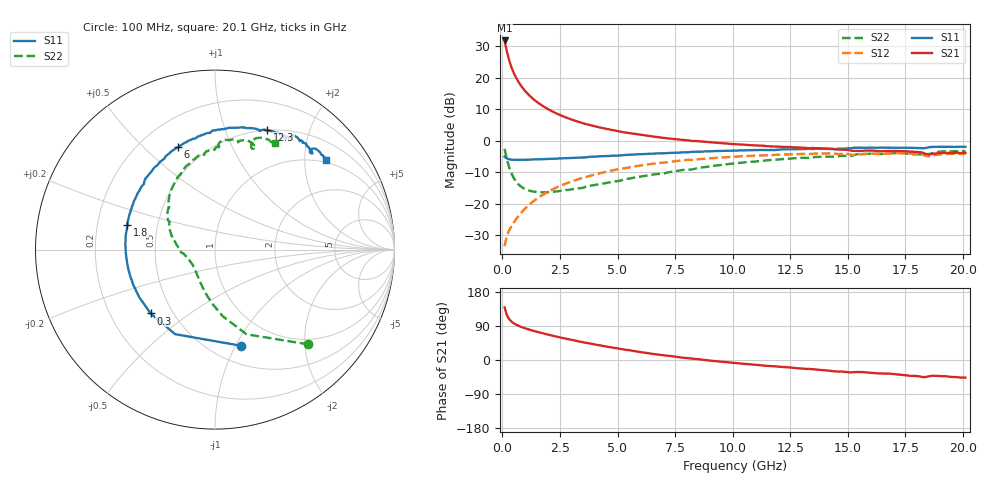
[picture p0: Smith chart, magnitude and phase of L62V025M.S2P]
!  Infineon Technologies AG
! BFR380L3 , PF131585-7, No.6, Th 09.10.01, soldered on pcb-board, measured with PP GSG850
!  Vce=2.0 V,  Ic=25.0 mA
! Common Emitter S-Parameters:  15. November 2001
#  GHz  S  MA  R  50
! f  S11  S21  S12  S22
! GHz  Mag  Ang  Mag  Ang  Mag  Ang  Mag  Ang
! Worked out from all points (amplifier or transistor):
!   201 points, 100 MHz to 20.1 GHz, reference 50 ohm
!   highest |S21| = 31.9 dB at 100 MHz (marker M1)
!   |S21| within 3 dB of that: start of sweep to 184.9 MHz
!   unconditionally stable (mu >= 1): 1.259 GHz to 4.37 GHz
!   at 3.4 GHz: K = 1.02, MAG = 8.1 dB, |S12| = -12.0 dB
!   at 10.1 GHz: K = 0.96, MSG = 2.0 dB, |S12| = -5.1 dB
!   at 20.1 GHz: K = 0.99, MSG = 0.2 dB, |S12| = -4.2 dB
!   S11 on the Smith chart (normalised r, x): 100 MHz: 0.68, -1.05; 300 MHz: 0.38, -0.36; 1.8 GHz: 0.33, +0.13; 6 GHz: 0.35, +0.64; 12.3 GHz: 0.50, +1.41; 20.1 GHz: 0.93, +2.54
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0.1  0.5554 -74.7  39.14 138.7  0.02101 63.4  0.7414 -45.4
0.2  0.521 -115.3  26.06 118.1  0.03068 54.9  0.5036 -69.6
0.3  0.5053 -135.3  18.82 107.8  0.03775 55.4  0.3732 -83.5
0.4  0.4984 -148.1  14.58 101.3  0.04361 56.9  0.299 -93.4
0.5  0.4958 -156.5  11.86 96.8  0.04995 59.4  0.2533 -101.2
0.6  0.4947 -162.8  9.981 93.3  0.0566 60.9  0.2234 -107.6
0.7  0.4951 -167.7  8.611 90.4  0.06321 62.2  0.2026 -113.3
0.8  0.4952 -171.8  7.569 87.8  0.07012 63.4  0.1879 -118.2
1  0.4973 -178.3  6.106 83.4  0.08409 64.6  0.1692 -126.6
1.2  0.5003 176.4  5.122 79.6  0.09809 65.3  0.1591 -133.4
1.5  0.504 169.6  4.133 74.4  0.1194 65.1  0.1522 -141.8
1.8  0.5076 164.0  3.472 69.7  0.1409 64.4  0.1507 -148.5
2.5  0.5214 152.2  2.558 59.7  0.19 61.1  0.1579 -160.6
3.5  0.5388 137.9  1.892 46.9  0.2578 54.8  0.1777 -173.3
4.6  0.5691 124.4  1.517 34.6  0.3266 47.4  0.2155 173.1
6  0.6085 109.7  1.24 20.8  0.4029 37.7  0.2687 158.0
6.8  0.6268 102.0  1.13 13.9  0.4418 31.8  0.2956 149.3
10.1  0.6972 77.8  0.8788 -7.9  0.556 10.3  0.4352 121.1
12.3  0.7274 66.5  0.7924 -18.9  0.6054 -3.0  0.5139 103.8
13.5  0.7356 60.7  0.7642 -24.5  0.6178 -9.9  0.5421 95.9
16.8  0.7728 48.4  0.6862 -35.9  0.6236 -25.5  0.6271 76.0
20.1  0.7961 38.8  0.6408 -46.4  0.618 -38.9  0.6822 60.5
